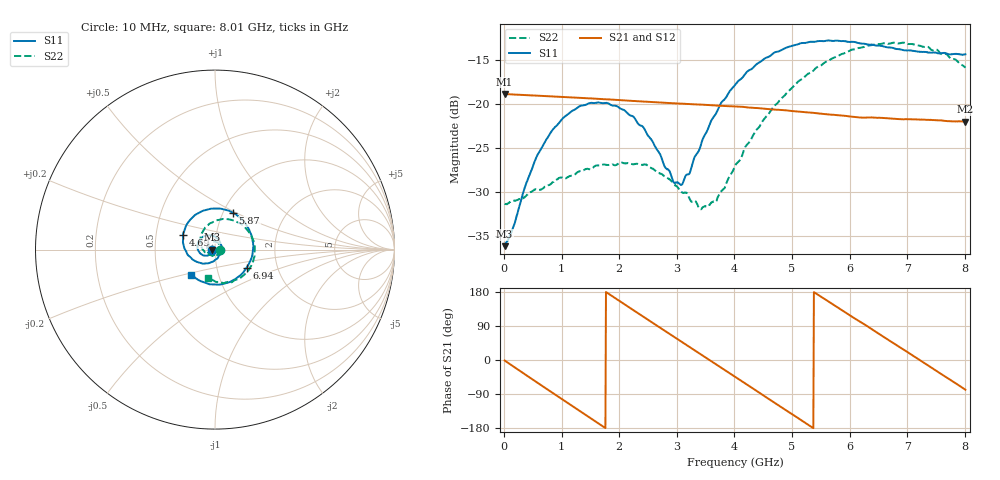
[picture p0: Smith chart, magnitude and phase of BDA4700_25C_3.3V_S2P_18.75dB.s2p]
!Agilent Technologies,E5071B,MY42404982,A.09.10
!Date: Mon Oct 20 18:10:55 2025
!Data & Calibration Information:
!Freq	S11:SOLT2(ON)	S21:SOLT2(ON)	S12:SOLT2(ON)	S22:SOLT2(ON)
# Hz S RI R 50
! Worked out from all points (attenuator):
!   801 points, 10 MHz to 8.01 GHz, reference 50 ohm
!   highest |S21| = -18.83 dB at 10 MHz (marker M1); lowest = -22.0 dB at 8 GHz (marker M2)
!   lowest |S11| = -36.2 dB at 10 MHz (marker M3), VSWR 1.03, Z = 48.5 - j0.114 ohm
!   |S11| at or under -10 dB: start of sweep to end of sweep
!   |S22| runs from -32.0 to -13.0 dB; largest |S21 - S12| = 0.0014
!   S11 on the Smith chart (normalised r, x): 10 MHz: 0.97, -0.00; 4.69 GHz: 0.69, +0.12; 5.87 GHz: 1.11, +0.48; 6.94 GHz: 1.39, -0.29; 8.01 GHz: 0.74, -0.21
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1e7  -0.0155 -0.00117  0.1144 -0.00248  0.1143 -0.00259  0.027 -0.000862
6e8  -0.0406 -0.0336  0.0524 -0.0986  0.0524 -0.0986  0.0129 -0.0298
1.01e9  -0.0788 -0.0243  -0.0261 -0.1068  -0.026 -0.1068  -0.0161 -0.0346
1.35e9  -0.098 0.0077  -0.0809 -0.0723  -0.0809 -0.0723  -0.0378 -0.0174
2.08e9  -0.0484 0.079  -0.0893 0.0554  -0.0893 0.0554  -0.0286 0.0361
2.42e9  -0.00172 0.0738  -0.0423 0.0944  -0.0423 0.0944  -0.002 0.0452
2.68e9  0.0259 0.0471  0.00319 0.1024  0.00306 0.1023  0.0162 0.0373
2.95e9  0.0351 0.00716  0.0485 0.0888  0.0483 0.0886  0.028 0.021
3.08e9  0.0323 -0.0128  0.067 0.0751  0.0663 0.0755  0.0299 0.0102
3.4e9  0.0021 -0.0561  0.0953 0.0285  0.0954 0.0286  0.0212 -0.0138
3.54e9  -0.0195 -0.0695  0.0988 0.00474  0.0988 0.0046  0.0125 -0.0231
3.69e9  -0.0477 -0.076  0.096 -0.0206  0.096 -0.0209  -0.0009 -0.0282
4.01e9  -0.1121 -0.0625  0.0697 -0.0675  0.0698 -0.0674  -0.0348 -0.0272
4.69e9  -0.1786 0.0814  -0.0351 -0.0862  -0.0348 -0.0864  -0.0828 0.0512
5.35e9  -0.0595 0.2183  -0.0893 -0.00331  -0.0892 -0.00392  -0.0139 0.1521
5.87e9  0.101 0.2052  -0.0565 0.065  -0.0564 0.0648  0.1062 0.1612
6.27e9  0.1893 0.1128  -0.00411 0.0836  -0.00283 0.0835  0.1891 0.0976
6.68e9  0.2092 -0.022  0.0507 0.0656  0.0509 0.0656  0.2207 -0.00693
6.94e9  0.1759 -0.1008  0.0729 0.0374  0.0732 0.037  0.2096 -0.0786
7.47e9  0.029 -0.1947  0.0735 -0.0344  0.0734 -0.0345  0.0996 -0.1775
8e9  -0.1299 -0.141  0.0173 -0.0776  0.0174 -0.0778  -0.0342 -0.1589
8.01e9  -0.1325 -0.1393  0.016 -0.078  0.0162 -0.0781  -0.0366 -0.1572
